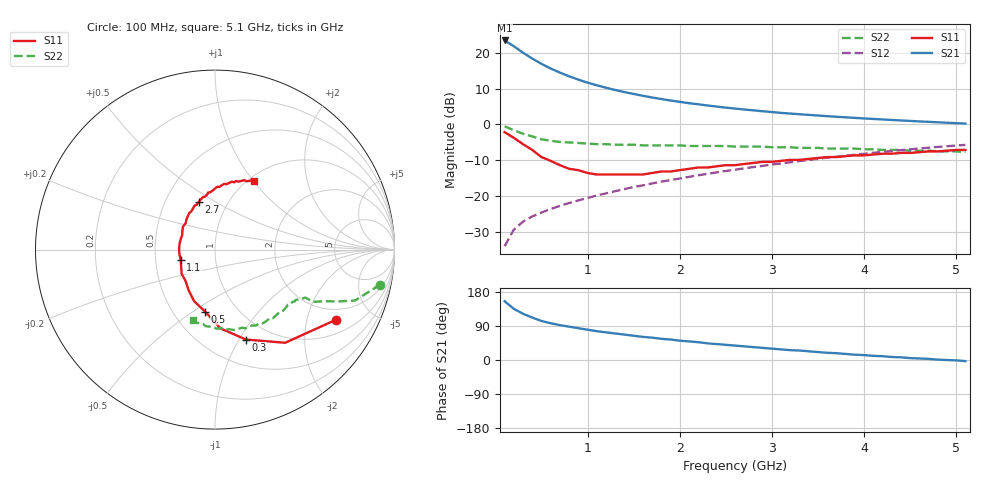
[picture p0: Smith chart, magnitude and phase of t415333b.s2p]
!AT-41533
!S and NOISE PARAMETERS at Vce=2.7V Ic=5mA. LAST UPDATED 01-25-95
# ghz s ma r 50
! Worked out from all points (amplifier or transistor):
!   51 points, 100 MHz to 5.1 GHz, reference 50 ohm
!   highest |S21| = 23.4 dB at 100 MHz (marker M1)
!   |S21| within 3 dB of that: start of sweep to 276.8 MHz
!   unconditionally stable (mu >= 1): 935.1 MHz to 2.414 GHz
!   at 900 MHz: K = 0.99, MSG = 16.9 dB, |S12| = -21.2 dB
!   at 2.6 GHz: K = 1.00, MSG = 8.5 dB, |S12| = -12.7 dB
!   at 5.1 GHz: K = 0.85, MSG = 3.0 dB, |S12| = -5.7 dB
!   lowest NFmin = 0.70 dB at 100 MHz
!   S11 on the Smith chart (normalised r, x): 100 MHz: 1.52, -3.03; 300 MHz: 0.77, -1.07; 500 MHz: 0.71, -0.56; 1.1 GHz: 0.67, -0.08; 2.7 GHz: 0.73, +0.42; 5.1 GHz: 1.07, +1.01
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0.1  0.78 -30.0  14.83 155.0  0.02 75.0  0.94 -12.0
0.2  0.65 -53.0  12.32 135.0  0.034 66.0  0.83 -20.0
0.3  0.53 -71.0  10.01 122.0  0.044 62.0  0.74 -23.0
0.4  0.44 -86.0  8.285 112.0  0.052 60.0  0.68 -25.0
0.5  0.35 -99.0  7.004 103.0  0.059 60.0  0.62 -28.0
0.6  0.31 -112.0  6.019 97.0  0.066 60.0  0.59 -28.0
0.7  0.27 -123.0  5.284 92.0  0.073 61.0  0.57 -28.0
0.8  0.24 -133.0  4.687 88.0  0.08 62.0  0.56 -29.0
1  0.21 -154.0  3.826 80.0  0.094 63.0  0.54 -31.0
1.1  0.2 -163.0  3.513 76.0  0.102 63.0  0.53 -32.0
1.3  0.2 178.0  3.021 70.0  0.117 64.0  0.52 -34.0
1.4  0.2 170.0  2.825 67.0  0.125 64.0  0.52 -35.0
1.6  0.2 156.0  2.508 61.0  0.141 64.0  0.51 -37.0
1.8  0.22 144.0  2.261 56.0  0.159 63.0  0.51 -40.0
2  0.23 134.0  2.065 51.0  0.176 63.0  0.51 -42.0
2.3  0.25 122.0  1.837 44.0  0.204 61.0  0.5 -47.0
2.6  0.27 112.0  1.663 38.0  0.233 59.0  0.49 -51.0
2.7  0.28 109.0  1.615 36.0  0.244 59.0  0.49 -53.0
3.1  0.31 98.0  1.447 28.0  0.285 55.0  0.48 -60.0
3.5  0.34 90.0  1.33 21.0  0.331 52.0  0.47 -69.0
4.3  0.39 74.0  1.153 8.0  0.425 43.0  0.44 -87.0
5.1  0.44 60.0  1.028 -3.0  0.518 32.0  0.41 -107.0
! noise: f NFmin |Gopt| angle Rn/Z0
0.1  0.7  0.45  8  0.2
0.9  1  0.25  94  0.13
1.8  1.4  0.38  -159  0.08
2.4  1.6  0.54  -122  0.16
